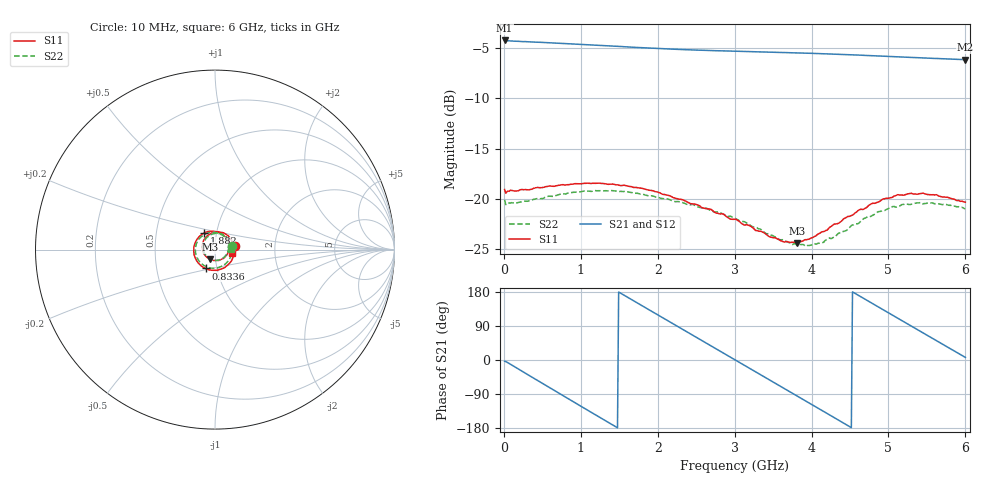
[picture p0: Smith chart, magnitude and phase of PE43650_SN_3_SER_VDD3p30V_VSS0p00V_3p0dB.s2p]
!Keysight Technologies,N5245B,MY57181451,A.13.50.07
!Date: Tuesday, May 07, 2019 07:59:50
!Correction: S11(Full 2 Port(1,2))
!S21(Full 2 Port(1,2))
!S12(Full 2 Port(1,2))
!S22(Full 2 Port(1,2))
!S2P File: Measurements: S11, S21, S12, S22:
# Hz S  dB  R 50
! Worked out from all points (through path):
!   401 points, 10 MHz to 6 GHz, reference 50 ohm
!   highest |S21| = -4.23 dB at 10 MHz (marker M1); lowest = -6.1 dB at 6 GHz (marker M2)
!   group delay of S21, straight-line fit = 329 ps
!   lowest |S11| = -24.4 dB at 3.814 GHz (marker M3), VSWR 1.13, Z = 47 - j5.06 ohm
!   |S11| at or under -10 dB: start of sweep to end of sweep
!   |S22| runs from -24.7 to -19.2 dB; largest |S21 - S12| = 0.0045
!   S11 on the Smith chart (normalised r, x): 10 MHz: 1.25, +0.05; 833.6 MHz: 0.88, -0.19; 1.882 GHz: 0.87, +0.16; 6 GHz: 1.21, -0.05
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1e7  -19.07 9.5  -4.23 -3.3  -4.28 -3.3  -20.09 12.8
2.34625e8  -19.08 -34.5  -4.34 -29.3  -4.39 -29.3  -20.27 -34.3
4.74225e8  -18.89 -68.6  -4.42 -58.4  -4.47 -58.4  -19.99 -68.2
8.33625e8  -18.58 -116.7  -4.55 -101.8  -4.60 -101.8  -19.43 -115.6
1.013325e9  -18.49 -139.4  -4.63 -123.4  -4.68 -123.4  -19.25 -137.3
1.4476e9  -18.60 170.5  -4.81 -175.3  -4.87 -175.3  -19.22 174.8
1.881875e9  -19.13 124.3  -4.99 133.2  -5.05 133.2  -19.70 131.3
2.01665e9  -19.38 110.8  -5.03 117.2  -5.09 117.2  -19.88 118.6
2.241275e9  -19.97 88.1  -5.11 90.7  -5.17 90.7  -20.28 97.4
2.4659e9  -20.51 64.8  -5.18 64.2  -5.23 64.3  -20.60 75.9
2.750425e9  -21.39 35.3  -5.25 30.7  -5.30 30.7  -21.30 47.5
3.005e9  -22.03 4.8  -5.30 0.7  -5.36 0.7  -21.91 19.9
3.45425e9  -23.78 -57.1  -5.40 -52.5  -5.44 -52.4  -23.54 -38.8
3.81365e9  -24.39 -117.3  -5.47 -95.0  -5.52 -95.0  -24.62 -95.3
4.008325e9  -23.86 -150.2  -5.52 -118.1  -5.56 -118.0  -24.56 -128.7
4.2629e9  -22.70 169.6  -5.58 -148.3  -5.64 -148.2  -23.94 -170.6
4.5025e9  -21.71 135.8  -5.65 -176.7  -5.71 -176.6  -22.79 152.8
4.7421e9  -20.65 105.1  -5.74 154.9  -5.79 155.1  -21.78 121.9
5.01165e9  -19.92 74.9  -5.82 123.1  -5.88 123.3  -20.89 89.9
5.4609e9  -19.47 30.3  -5.97 70.2  -6.02 70.3  -20.47 45.6
5.745425e9  -19.84 6.7  -6.06 36.7  -6.11 36.8  -20.55 21.4
6e9  -20.33 -11.6  -6.14 6.8  -6.19 6.9  -20.98 3.2
